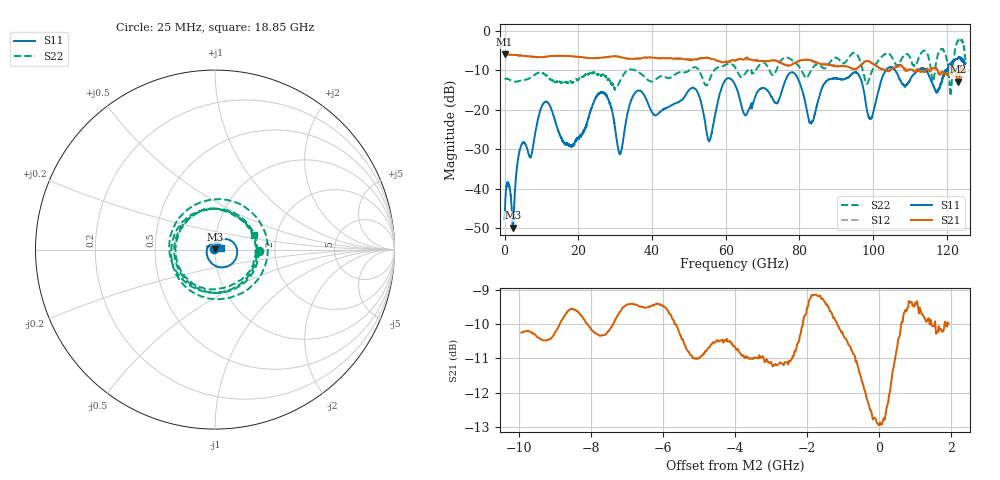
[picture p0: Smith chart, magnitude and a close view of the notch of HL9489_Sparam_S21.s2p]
! 2/28/2024 4:14:49 PM
! H:\PROTOTYPE_DATA\2-2024-110GHZ\4A-S21.S2P
! CHANNEL.1
! TR.MEASUREMENT
! CORRECTED.DATA
# GHZ S RI R 50.0
! FREQ.GHZ  S11RE  S11IM  S21RE  S21IM  S12RE  S12IM  S22RE  S22IM
!; PortSelection: Port_12
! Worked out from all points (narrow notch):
!   5000 points, 25 MHz to 125 GHz, reference 50 ohm
!   highest |S21| = -5.98 dB at 25 MHz (marker M1); lowest = -13.0 dB at 123.1 GHz (marker M2)
!   notch at M2: 5.5 dB deep, 1.65 GHz wide at half that depth
!   lowest |S11| = -49.8 dB at 2.35 GHz (marker M3), VSWR 1.01, Z = 50.2 + j0.273 ohm
!   |S11| at or under -10 dB: start of sweep to 103.5 GHz; 105.9 GHz to 112.3 GHz (6.385 GHz wide, 5.85 % of centre); 114.4 GHz to 119.9 GHz (5.516 GHz wide, 4.71 % of centre)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
!   |S22| runs from -16.2 to -2.2 dB; largest |S21 - S12| = 0.14
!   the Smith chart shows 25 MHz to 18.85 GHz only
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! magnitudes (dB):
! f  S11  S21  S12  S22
! 25 MHz  -47.7  -6.0  -6.0  -12.3
! 2.35 GHz  -49.8  -6.1  -6.1  -12.8
! 4.325 GHz  -29.6  -6.3  -6.3  -12.6
! 10.7 GHz  -18.2  -6.7  -6.6  -11.0
! 20.88 GHz  -26.3  -6.7  -6.7  -11.8
! 26.12 GHz  -15.7  -6.8  -6.9  -11.4
! 31.27 GHz  -31.3  -6.7  -6.7  -12.9
! 35.62 GHz  -15.5  -7.1  -7.1  -10.1
! 41.7 GHz  -21.0  -7.0  -7.0  -11.8
! 51.42 GHz  -14.6  -7.3  -7.4  -9.3
! 55.55 GHz  -28.0  -6.9  -6.9  -12.6
! 62.52 GHz  -13.7  -7.6  -7.5  -9.3
! 65.4 GHz  -21.4  -6.9  -7.3  -10.7
! 78.33 GHz  -10.6  -8.4  -8.3  -7.7
! 83.35 GHz  -23.2  -7.6  -7.7  -9.8
! 95.03 GHz  -10.5  -9.8  -9.7  -5.7
! 99.33 GHz  -22.3  -8.1  -8.0  -11.0
! 104.2 GHz  -9.4  -10.3  -10.0  -5.8
! 118.8 GHz  -12.1  -10.5  -10.9  -4.7
! 121 GHz  -8.4  -9.9  -10.2  -16.2
! 123.1 GHz  -6.8  -13.0  -10.9  -2.5
! 125 GHz  -8.2  -10.0  -9.5  -7.5
